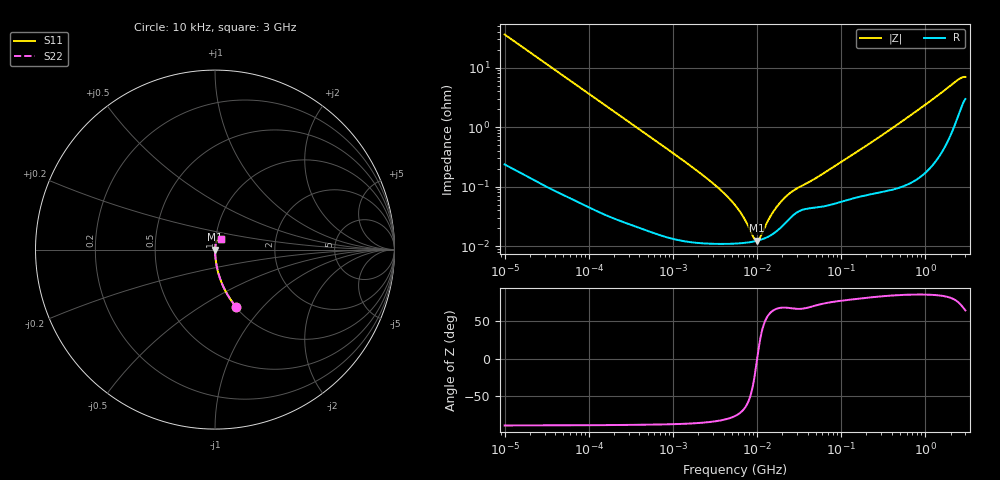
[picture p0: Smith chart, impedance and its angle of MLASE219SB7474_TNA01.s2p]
! MLASE219SB7474_TNA01  S-PARAMETER MODEL  ( Standard Model )
! Model Generated by TAIYO YUDEN Corporation (http://www.ty-top.com)
! Version 2.0
! TAIYO YUDEN Control No. 240510
! Copyright(c) 2009 TAIYO YUDEN CO.,LTD. All Rights Reserved.
! Product Description (link to TY-COMPAS)
! https://ds.yuden.co.jp/TYCOMPAS/or/detail?pn=MLASE219SB7474KTNA01&u=M
! Products Name : Multilayer Ceramic Capacitors
! Characteristics :
!  Capacitance : 0.47 [uF] , Rated Voltage : 16 [V] , TCC : X7R
!  Case Size : 2.0 x 1.25 / 0.079 x 0.049 [mm/inch] , Thickness : 0.85 / 0.033 [mm/inch]
!  (Conditions: Temperature = 25 [degC] , DC Bias Voltage = 0 [V])
! External Node Assignments :
!  1  o---| |---o  2
! GND o---------o GND
! Frequency Range : 10kHz  -  3GHz  [ 401 STEP ]
# MHZ S RI R 50
! Freq[MHz].  S11 Real  S11 Imag  S21 Real  S21 Imag  S12 Real  S12 Imag  S22 Real  S22 Imag
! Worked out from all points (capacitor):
!   401 points, 10 kHz to 3 GHz, reference 50 ohm
!   read as one part in series: C = 440 nF near 10.65 kHz
!   lowest |Z| = 12.3 mohm at 9.971 MHz (marker M1)
!   series resonance near 10.05 MHz, so ESL is about 570 pH
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0.01  0.117 -0.3182  0.883 0.3182  0.883 0.3182  0.117 -0.3182
0.015549  0.0528 -0.2201  0.9472 0.2201  0.9472 0.2201  0.0528 -0.2201
0.026575  0.0194 -0.1337  0.9806 0.1337  0.9806 0.1337  0.0194 -0.1337
0.082683  0.00246 -0.044  0.9975 0.044  0.9975 0.044  0.00246 -0.044
0.683653  0.000184 -0.0054  0.9998 0.0054  0.9998 0.0054  0.000184 -0.0054
2.737278  0.000112 -0.00126  0.9999 0.00126  0.9999 0.00126  0.000112 -0.00126
4.124064  0.00011 -0.000753  0.9999 0.000753  0.9999 0.000753  0.00011 -0.000753
5.477226  0.000111 -0.00048  0.9999 0.00048  0.9999 0.00048  0.000111 -0.00048
7.048603  0.000114 -0.00027  0.9999 0.00027  0.9999 0.00027  0.000114 -0.00027
9.070798  0.00012 -7.66e-05  0.9999 7.66e-05  0.9999 7.66e-05  0.00012 -7.66e-05
9.97066  0.000123 -5.63e-06  0.9999 5.63e-06  0.9999 5.63e-06  0.000123 -5.63e-06
10.95979  0.000128 6.56e-05  0.9999 -6.56e-05  0.9999 -6.56e-05  0.000128 6.56e-05
13.24217  0.000142 0.000211  0.9999 -0.000211  0.9999 -0.000211  0.000142 0.000211
15.50326  0.000161 0.000337  0.9998 -0.000337  0.9998 -0.000337  0.000161 0.000337
19.95104  0.000218 0.00055  0.9998 -0.00055  0.9998 -0.00055  0.000218 0.00055
27.34599  0.000338 0.0008  0.9997 -0.0008  0.9997 -0.0008  0.000338 0.0008
45.28751  0.00044 0.0012  0.9996 -0.0012  0.9996 -0.0012  0.00044 0.0012
374.4521  0.000943 0.00886  0.9991 -0.00886  0.9991 -0.00886  0.000943 0.00886
1026.989  0.00235 0.0243  0.9976 -0.0243  0.9976 -0.0243  0.00235 0.0243
2405.867  0.0173 0.0579  0.9827 -0.0579  0.9827 -0.0579  0.0173 0.0579
2729.247  0.0261 0.0614  0.9739 -0.0614  0.9739 -0.0614  0.0261 0.0614
3000  0.0326 0.0594  0.9674 -0.0594  0.9674 -0.0594  0.0326 0.0594
